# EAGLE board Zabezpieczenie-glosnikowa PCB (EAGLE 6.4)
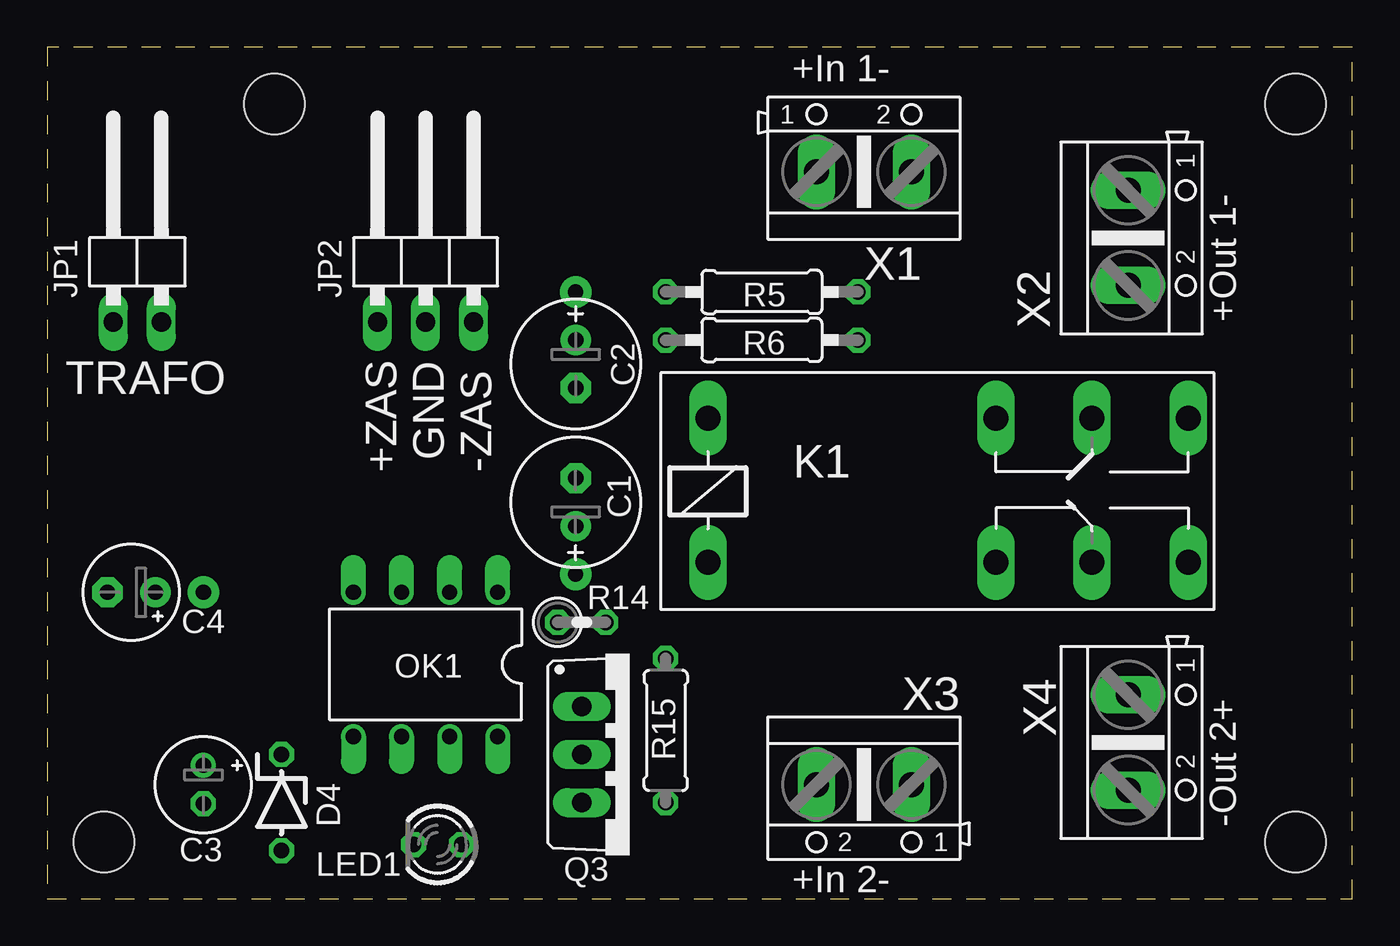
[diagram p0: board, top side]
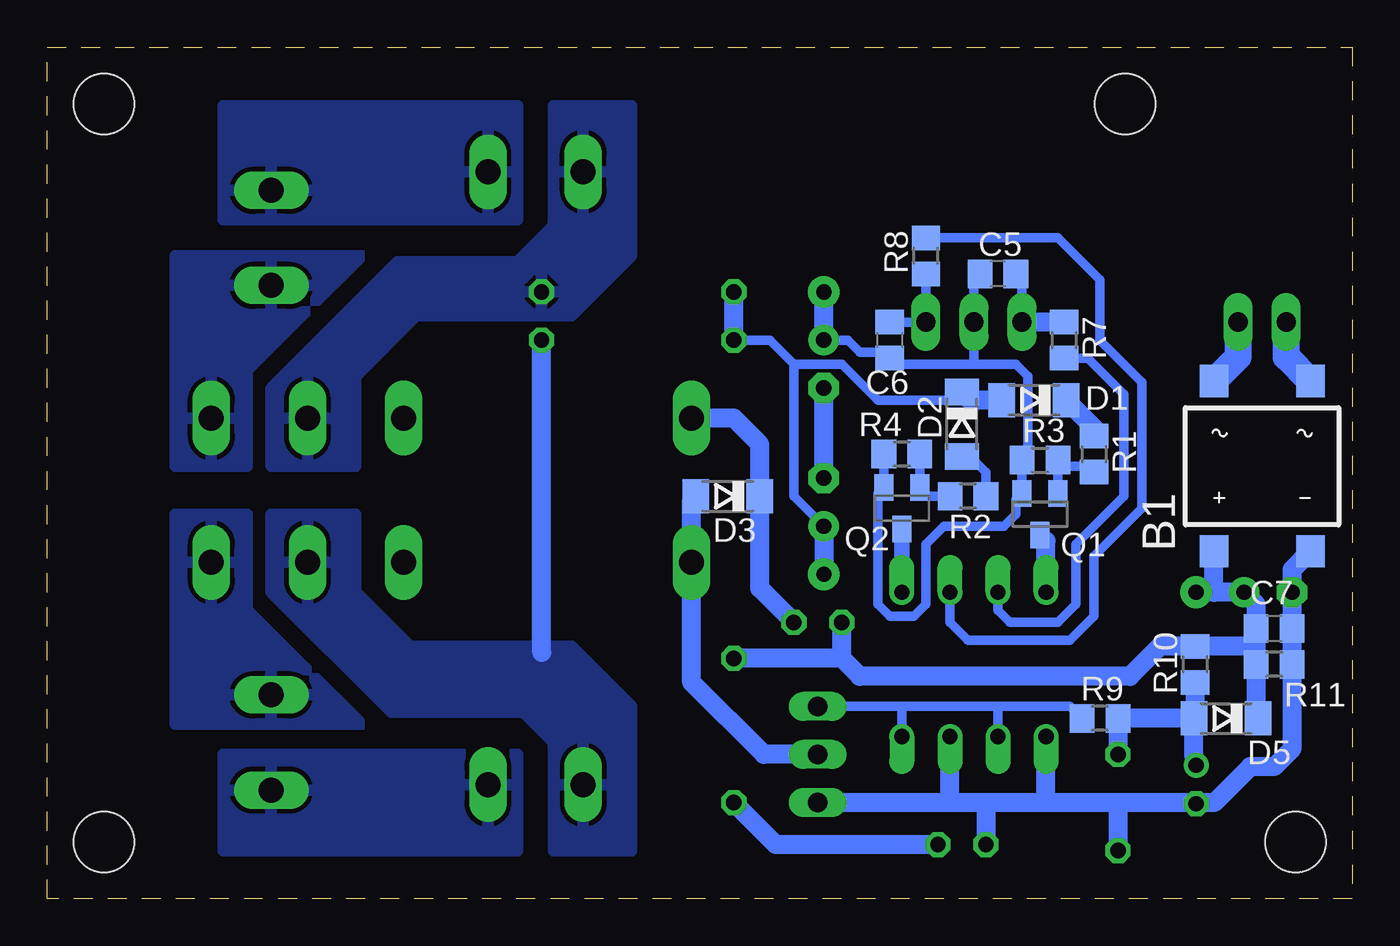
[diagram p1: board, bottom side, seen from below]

Size 69 x 45 mm. Coordinates in mm from the lower left corner, seen from the top.
Outline: 0,0 69,0 69,45 0,45 0,0
Copper layers (1*16): Top 0.035mm / dielectric 1.5mm / Bottom 0.035mm
Design rules "AVT-Elmax": minimum track width 8mil, minimum drill 18mil, track to track 8mil, track to pad 8mil, pad to pad 8mil, via to via 8mil, smd to smd 8mil, copper to edge 10mil, drill to drill 8mil, minimum pad ring 10mil, minimum via ring 8mil, stop-mask expansion 4mil, vias tented up to drill 0mil, thermal gap 10mil
Holes 3.2 mm at 3,3 12,42 66,42 66,3

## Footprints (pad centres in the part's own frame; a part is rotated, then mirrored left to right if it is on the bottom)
DFS = smd 1.5 x 1.7: + -2.55,-4.5; - 2.55,-4.5; AC1 -2.55,4.5; AC2 2.55,4.5
E2,5-7 = drill 0.813 pad 1.6: + -1.27,0 | drill 0.813 pad 1.6 octagon: - 1.27,0
E2-5 = drill 0.813 pad 1.27: + -1.016,0 | drill 0.813 pad 1.27 octagon: - 1.016,0
E2,5-5 = drill 0.813 pad 1.6: + -1.27,0 | drill 0.813 pad 1.6 octagon: - 1.27,0
C0805 = smd 1.3 x 1.5: 1 -0.95,0; 2 0.95,0
SOD80C = smd 1.4 x 1.8: A 1.7,0; C -1.7,0
ZDIO-5 = drill 0.813 octagon: A 2.54,0; C -2.54,0
1X02/90 = drill 1.016 long: 1 -1.27,-3.81; 2 1.27,-3.81
1X03/90 = drill 1.016 long: 1 -2.54,-3.81; 2 0,-3.81; 3 2.54,-3.81
F4052 = drill 1.321 long: 1 -3.81,3.81; 2 -3.81,-3.81; O1 11.43,-3.81; O2 11.43,3.81; P1 16.51,-3.81; P2 16.51,3.81; S1 21.59,-3.81; S2 21.59,3.81
LED3MM = drill 0.813 octagon: A -1.27,0; K 1.27,0
DIL08 = drill 0.813 offset: 1 -3.81,-3.81; 2 -1.27,-3.81; 3 1.27,-3.81; 4 3.81,-3.81; 5 3.81,3.81; 6 1.27,3.81; 7 -1.27,3.81; 8 -3.81,3.81
SOT23 = smd 1 x 1.4: 1 -0.95,-1.1; 2 0.95,-1.1; 3 0,1.1
SOT23-BEC = smd 1 x 1.4: B -0.95,-1.1; C 0,1.1; E 0.95,-1.1
TO220BV = drill 1.016 long: D 0,-2.54; G -2.54,-2.54; S 2.54,-2.54
R0805 = smd 1.3 x 1.5: 1 -0.95,0; 2 0.95,0
0207/10 = drill 0.813 octagon: 1 -5.08,0; 2 5.08,0
0207/2V = drill 0.813 octagon: 1 -1.27,0; 2 1.27,0
0207/7 = drill 0.813 octagon: 1 -3.81,0; 2 3.81,0
AK500/2 = drill 1.321 long: 1 -2.515,0; 2 2.515,0

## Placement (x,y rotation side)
B1  DF06S  [DFS]  4.76,22.86 0 bottom
C1  47u  [E2,5-7]  27.94,20.95 90 top
C2  47u  [E2,5-7]  27.94,28.26 270 top
C3  10u  [E2-5]  8.26,6.03 270 top
C4  47u  [E2,5-5]  4.45,16.19 180 top
C5  100n  [C0805]  18.73,33.02 180 bottom
C6  100n  [C0805]  24.45,29.53 90 bottom
C7  100n  [C0805]  4.13,14.29 0 bottom
D1  1N4148  [SOD80C]  16.83,26.35 180 bottom
D2  1N4148  [SOD80C]  20.64,25.08 270 bottom
D3  1N4148  [SOD80C]  33.02,21.27 180 bottom
D4  15V  [ZDIO-5]  12.38,5.08 270 top
D5  1N4148  [SOD80C]  6.67,9.53 180 bottom
JP1  Trafo  [1X02/90]  4.76,34.29 0 top
JP2  Zasilanie  [1X03/90]  20,34.29 0 top
K1  RM84  [F4052]  38.73,21.59 0 top
LED1  [LED3MM]  20.64,2.86 180 top
OK1  LTV826  [DIL08]  20,12.38 180 top
Q1  BC846  [SOT23]  16.51,20.32 180 bottom
Q2  BC858  [SOT23-BEC]  23.81,20.64 180 bottom
Q3  IRF520  [TO220BV]  30.8,7.62 270 top
R1  33k  [R0805]  13.65,23.5 270 bottom
R2  33k  [R0805]  20.32,21.27 180 bottom
R3  *  [R0805]  16.51,23.18 0 bottom
R4  *  [R0805]  23.81,23.5 180 bottom
R5  22k  [0207/10]  37.78,32.07 180 top
R6  22k  [0207/10]  37.78,29.53 180 top
R7  4k7  [R0805]  15.24,29.53 270 bottom
R8  4k7  [R0805]  22.54,33.97 90 bottom
R9  4k7  [R0805]  13.34,9.53 180 bottom
R10  1M  [R0805]  8.3,12.38 90 bottom
R11  4k7  [R0805]  4.13,12.38 180 bottom
R14  *  [0207/2V]  28.26,14.61 0 top
R15  RLED  [0207/7]  32.7,8.89 90 top
X1  [AK500/2]  43.18,38.42 0 top
X2  [AK500/2]  57.15,34.92 270 top
X3  [AK500/2]  43.18,6.03 180 top
X4  [AK500/2]  57.15,8.26 270 top

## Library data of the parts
B1 = rectifier
C1-C7 R1-R11 R14 R15 = rcl
D1-D5 = diode
JP1 JP2 = pinhead
K1 = relay; OC_FARNELL: unknown; OC_NEWARK: unknown
LED1 = led
OK1 = optocoupler; OC_FARNELL: unknown; OC_NEWARK: unknown
Q1 = transistor-npn
Q2 = transistor-pnp
Q3 = transistor-power
X1-X4 = con-ptr500; OC_FARNELL: unknown; OC_NEWARK: unknown

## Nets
GND: C2.+ C5.2 C6.1 JP2.2 Q1.2 Q2.E R3.1 R4.2
N$1: D1.C R1.1
N$2: Q1.1 R1.2 R3.2
N$3: Q2.B R2.2 R4.1
N$4: OK1.2 R8.2
N$5: D2.A R2.1
N$6: D3.A K1.2 Q3.D
N$7: C1.- C2.-
N$8: OK1.1 Q2.C
N$9: OK1.3 R7.2
N$10: OK1.4 Q1.3
N$11: K1.P1 R6.1 X3.2
N$12: B1.+ C4.+ C7.1 D5.C R10.2 R11.2 R14.1 R15.2
N$13: OK1.6 OK1.8 Q3.G R9.2
N$14: B1.- C3.- C4.- C7.2 D4.A LED1.K OK1.5 OK1.7 Q3.S R11.1
N$15: C3.+ D4.C D5.A R9.1 R10.1
N$16: C1.+ D1.A D2.C R5.2 R6.2
N$17: K1.P2 R5.1 X1.1
N$18: B1.AC2 JP1.1
N$19: B1.AC1 JP1.2
N$20: X1.2 X2.1
N$21: K1.S2 X2.2
N$22: K1.S1 X4.1
N$23: X3.1 X4.2
N$25: D3.C K1.1 R14.2
N$26: LED1.A R15.1
VCC: C5.1 JP2.1 R7.1
VSS: C6.2 JP2.3 R8.1

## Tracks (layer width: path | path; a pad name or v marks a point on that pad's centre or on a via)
GND  (via drill 0.8 pad 1.68)
  Bottom 0.508: Q2.E R4.2 | Q2.E 24.76,21.59 | Q2.E 25.08,21.42 25.08,15.56 24.45,14.92 23.18,14.92 22.54,15.56 22.54,18.73 21.59,19.68 18.41,19.68 17.78,20.32 17.78,21.1 Q1.2 R3.1 17.14,23.49 17.14,27.62 17.78,28.26 20,28.26 | 20,28.26 JP2.2 20,32.7 C5.2 | 20,28.26 24.13,28.26 C6.1 24.76,28.89 26.04,28.89 26.67,29.53 C2.+
  Bottom 1.016: C2.+ v27.94,32.07
N$1
  Bottom 1.016: R1.1 13.65,24.88 D1.C
N$2
  Bottom 0.508: 15.56,21.91 Q1.1 | 15.56,21.91 R3.2 15.24,22.86 13.97,22.86 R1.2 | 15.56,21.91
N$3
  Bottom 0.508: R4.1 Q2.B 22.4,21.27 R2.2
N$4
  Bottom 0.508: OK1.2 21.27,14.61 20.32,13.65 14.92,13.65 13.65,14.92 13.65,18.1 11.11,20.64 11.11,27.3 13.34,29.53 13.34,32.7 15.55,34.92 R8.2
N$5
  Bottom 0.508: R2.1 19.37,22.55 20.21,23.38 D2.A
N$6
  Bottom 1.016: Q3.D 31.11,7.62 34.92,11.43 K1.2 34.92,21.07 D3.A
N$7
  Bottom 1.016: C1.- C2.-
N$8
  Bottom 0.813: OK1.1 Q2.C
N$9
  Bottom 0.508: OK1.3 18.73,15.24 18.1,14.61 15.56,14.61 14.61,15.56 14.61,18.73 12.06,21.27 12.06,26.67 13.97,28.57 R7.2
N$10
  Bottom 1.016: Q1.3 16.19,18.9 OK1.4
N$11
  Bottom 1.016: 42.86,13.02 R6.1
  pour Bottom: 57.15,20.32 57.15,16.19 50.8,9.84 43.81,9.84 42.23,8.26 42.23,2.54 38.1,2.54 38.1,10.16 41.27,13.34 49.85,13.34 52.7,16.19 52.7,20.32
N$12  (via drill 0.8 pad 1.68)
  Bottom 1.016: R11.2 C7.1 5.08,15.55 C4.+ 7.3,16.19 | R11.2 5.08,13.33 R10.2 10.16,13.33 11.75,11.75 26.04,11.75 26.99,12.7 | R11.2 5.08,9.63 D5.C | 26.99,12.7 R15.2 | 26.99,12.7 R14.1 | 7.3,16.19 v8.26,16.19 | B1.+ 7.31,16.2 7.3,16.19
N$13
  Bottom 0.508: 18.73,10.16 OK1.6 | 18.73,10.16 14.92,10.16 R9.2 | 18.73,10.16 23.81,10.16 | 23.81,10.16 Q3.G | 23.81,10.16 OK1.8
N$14
  Bottom 1.016: 8.26,5.08 7.3,5.08 5.4,6.99 4.13,6.99 3.18,7.93 R11.1 C7.2 3.18,16 C4.- 3.17,17.4 B1.- | 8.26,5.08 C3.- | 8.26,5.08 12.38,5.08 | 12.38,5.08 16.19,5.08 | 16.19,5.08 19.37,5.08 | 19.37,5.08 21.27,5.08 | 21.27,5.08 Q3.S | 21.27,5.08 OK1.7 | 16.19,5.08 OK1.5 | 12.38,5.08 D4.A | 19.37,5.08 LED1.K
N$15
  Bottom 1.016: D4.C R9.1 D5.A | D5.A 8.37,7.48 C3.+ | R10.1 8.3,9.59 D5.A
N$16  (via drill 0.8 pad 1.68)
  Bottom 0.508: D2.C 21.07,26.35 25.08,26.35 26.99,28.26 29.53,28.26 | C1.+ 29.53,21.27 29.53,28.26 | R6.2 30.8,29.53 29.53,28.26
  Bottom 1.016: D1.A 20.21,26.35 D2.C | R6.2 R5.2 | C1.+ v27.94,17.14
N$17
  pour Bottom: 42.23,41.91 42.23,35.56 44.13,33.66 50.48,33.66 57.15,26.99 57.15,22.86 52.7,22.86 52.7,27.62 49.53,30.8 41.27,30.8 38.1,33.97 38.1,41.91
N$18
  Bottom 1.422: JP1.1 3.49,28.64 B1.AC2
N$19
  Bottom 1.422: JP1.2 6.03,28.64 B1.AC1
N$20
  pour Bottom: 44.13,41.91 44.13,35.88 59.69,35.88 59.69,41.91
N$21
  pour Bottom: 58.42,22.86 58.42,27.94 52.39,33.97 62.23,33.97 62.23,22.86
N$22
  pour Bottom: 52.39,9.21 62.23,9.21 62.23,20.32 58.42,20.32 58.42,15.24
N$23
  pour Bottom: 59.69,7.62 44.13,7.62 44.13,2.54 59.69,2.54
N$25
  Bottom 1.016: K1.1 32.7,25.4 31.32,24.02 D3.C 31.32,16.4 R14.2
N$26
  Bottom 1.016: LED1.A 30.48,2.86 R15.1
VCC
  Bottom 0.508: JP2.1 17.46,32.7 C5.1
  Bottom 1.016: R7.1 JP2.1
VSS
  Bottom 0.508: R8.1 JP2.3 C6.2

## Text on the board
tPlace: +In 1- | +Out 1- | TRAFO | +ZAS / GND / -ZAS | -Out 2+ | +In 2-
